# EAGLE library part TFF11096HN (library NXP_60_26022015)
Low phase noise LO generator for VSAT applications The TFF11096HN is a Ku band frequency generator intended for low phase noise Local Oscillator (LO) circuits for Ku band VSAT transmitters and transceivers. The specified phase noise complies with IESS-308 from Intelsat. AAL Eindhoven MK
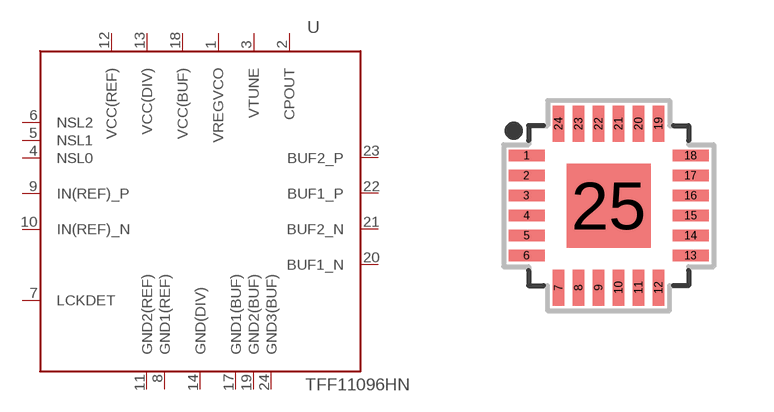
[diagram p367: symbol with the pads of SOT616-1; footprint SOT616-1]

Designator prefix U

## TFF11096HN  [SOT616-1]
1  VREGVCO  pas
2  CPOUT  pas
3  VTUNE  pas
4  NSL0  in
5  NSL1  in
6  NSL2  in
7  LCKDET  in
8  GND1(REF)  pwr
9  IN(REF)_P  in
10  IN(REF)_N  in
11  GND2(REF)  pwr
12  VCC(REF)  pwr
13  VCC(DIV)  pwr
14  GND(DIV)  pwr
17  GND1(BUF)  pwr
18  VCC(BUF)  pwr
19  GND2(BUF)  pwr
20  BUF1_N  out
21  BUF2_N  out
22  BUF1_P  out
23  BUF2_P  out
24  GND3(BUF)  pwr

## Footprint SOT616-1 (pad centres in mm)
SOT616-1 HVQFN24: plastic thermal enhanced very thin quad flat package; no leads; 24 terminals; body 4 x 4 x 0.85 mm JEDEC: MO-220 IEC: -- JEITA: --
smd 0.9 x 0.29: 1 -2.05,1.25; 2 -2.05,0.75; 3 -2.05,0.25; 4 -2.05,-0.25; 5 -2.05,-0.75; 6 -2.05,-1.25; 13 2.05,-1.25; 14 2.05,-0.75; 15 2.05,-0.25; 16 2.05,0.25; 17 2.05,0.75; 18 2.05,1.25
smd 0.29 x 0.9: 7 -1.25,-2.05; 8 -0.75,-2.05; 9 -0.25,-2.05; 10 0.25,-2.05; 11 0.75,-2.05; 12 1.25,-2.05; 19 1.25,2.05; 20 0.75,2.05; 21 0.25,2.05; 22 -0.25,2.05; 23 -0.75,2.05; 24 -1.25,2.05
smd 2.1 x 2.1: 25 0,0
